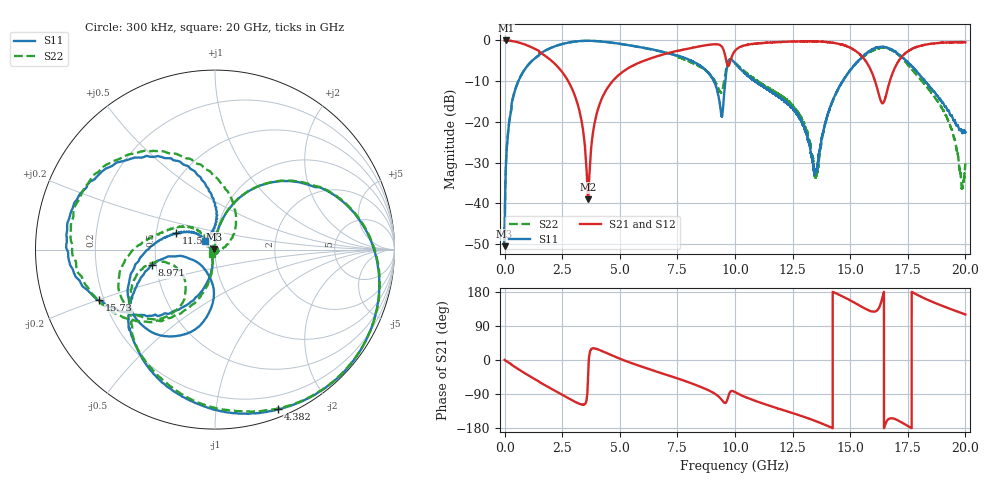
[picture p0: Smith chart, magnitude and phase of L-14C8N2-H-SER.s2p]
!{L-14C8N2}
!Johanson Technology Inc.
!www.johansontechnology.com
!Test Board Conditions:
!Substrate Type  RO4350B
!Substrate Thickness  20 mil
!Substrate Dk  3.66
!TL Type: GCPW
!TL Trace Width  36 mil
!TL Gap  12 mil
!Electrode orientation  Horizontal
!DUT TOPOLOGY	SERIES
!Mounting Pad LxW  26x36 mil
! Created Sun Jun 20 12:59:43 2021
# hz S ma R 50
! 2 Port Network Data from SP1.SP block
! freq  magS11  angS11  magS21  angS21  magS12  angS12  magS22  angS22
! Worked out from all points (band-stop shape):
!   20001 points, 300 kHz to 20 GHz, reference 50 ohm
!   highest |S21| = -0.01 dB at 52.3 MHz (marker M1); lowest = -39.0 dB at 3.624 GHz (marker M2)
!   |S21| within 3 dB of the highest: 9.943 GHz to 15.34 GHz (5.399 GHz wide, 42.7 % of centre); 17.42 GHz to end of sweep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
!   lowest |S11| = -50.5 dB at 1.3 MHz (marker M3), VSWR 1.01, Z = 49.7 + j0.0824 ohm
!   |S11| at or under -10 dB: start of sweep to 598.1 MHz; 10.87 GHz to 14.67 GHz (3.8 GHz wide, 29.8 % of centre); 18.25 GHz to end of sweep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
!   |S22| runs from -50.4 to -0.1 dB; largest |S21 - S12| = 0.014
!   S11 on the Smith chart (normalised r, x): 300 kHz: 0.99, -0.00; 4.382 GHz: 0.07, -1.47; 8.971 GHz: 0.48, -0.09; 11.55 GHz: 0.64, +0.12; 15.73 GHz: 0.18, -0.20; 20 GHz: 0.89, +0.09
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300000  0.004983 -164.0  0.9957 0.2  0.9946 0.2  0.005014 -162.0
1300000  0.002976 163.8  0.9971 0.0  0.9972 0.0  0.003031 157.7
5.23e7  0.02697 90.0  0.999 -2.1  0.9979 -2.1  0.02701 90.2
2.723e8  0.1328 79.5  0.9904 -10.6  0.9903 -10.5  0.1341 79.5
7.383e8  0.3811 59.6  0.9188 -29.6  0.92 -29.6  0.3827 59.7
2.2393e9  0.8583 5.5  0.4966 -82.9  0.4965 -82.9  0.8566 6.2
3.3343e9  0.9845 -33.9  0.105 -117.3  0.1053 -117.3  0.9833 -32.2
3.6243e9  0.9899 -44.0  0.01122 -42.0  0.01122 -42.7  0.9876 -42.4
4.3823e9  0.9571 -68.4  0.2388 19.8  0.2394 19.6  0.9589 -66.0
6.6673e9  0.7476 -120.8  0.6449 -32.1  0.6462 -31.9  0.7423 -120.0
8.9713e9  0.3598 -166.3  0.8906 -83.6  0.8892 -83.8  0.3688 -167.8
9.4163e9  0.1183 -140.1  0.8461 -104.5  0.8499 -104.6  0.2302 -140.2
9.7053e9  0.5403 -116.3  0.4843 -97.2  0.4888 -97.1  0.5534 -137.2
1.00003e10  0.5264 -156.8  0.7442 -84.6  0.7469 -84.6  0.5345 -168.7
1.15513e10  0.2344 157.2  0.9433 -121.7  0.944 -121.8  0.2524 151.0
1.33343e10  0.03708 148.1  0.9757 -157.5  0.9745 -157.5  0.03954 138.5
1.35343e10  0.02572 -139.8  0.9732 -162.1  0.97 -162.1  0.02219 -155.3
1.42663e10  0.1906 -103.6  0.9335 179.4  0.9361 179.3  0.1875 -101.1
1.57313e10  0.704 -156.3  0.5277 132.9  0.5315 132.5  0.6863 -152.2
1.66673e10  0.7962 154.6  0.2812 -155.9  0.276 -154.3  0.798 149.9
1.80053e10  0.3816 99.2  0.851 169.1  0.8562 169.4  0.3418 80.3
2e10  0.07494 139.4  0.9528 120.1  0.9482 120.0  0.03098 -125.3
